PROGRAM MAIN
(* The project need a CX7000 with Image 140501 or higher, NTP Server is in the project ntp.beckhoff.com -> use here a locel or own NTP Server

The example read the NTP Time check the status, show this via digital Output and WD LED 
And let a LED flashing very sec
// Toggle Outpt every Sec
IF (sec_1 MOD 2) =0 THEN
	gvl.bCX7028_Out_4:=TRUE;
ELSE
	gvl.bCX7028_Out_4:=FALSE;
END_IF

If you have a second CX7000 you can see and measurement the differnts between the both CX7000.

*) 
VAR
END_VAR

TimeSync();

END_PROGRAM
